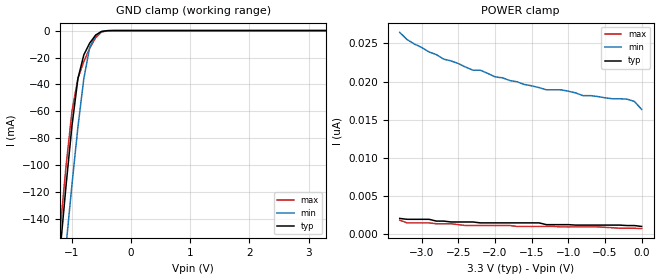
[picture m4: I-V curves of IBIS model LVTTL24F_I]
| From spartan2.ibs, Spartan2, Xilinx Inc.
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|   Model LVTTL24F_I
[Model]   LVTTL24F_I
Model_type   Input
Polarity   Non-Inverting
Vinl =   0.800V
Vinh =   2.000V
C_comp   6.5000pF   5.0000pF   8.0000pF
[Temperature Range]   27.0000   100.0000   0.000
[Voltage Range]   3.3000V   3.0000V   3.6000V
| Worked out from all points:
|   GND clamp passes 1 mA (typ) near -0.51 V on its own axis
[GND_clamp]
| voltage   I(typ)   I(min)   I(max)
-3.3V     -1.286A    -1.273A    -1.29A
-1.3V     -213.2mA   -255.1mA   -198mA
-1.2V     -163mA     -206.8mA   -147.7mA
-1.1V     -114.8mA   -159.6mA   -100.3mA
-1V       -70.57mA   -114.1mA   -59.86mA
-900mV    -35.79mA   -71.75mA   -35.46mA
-800mV    -18.04mA   -35.69mA   -22.98mA
-700mV    -9.256mA   -12.38mA   -13.06mA
-600mV    -3.388mA   -3.468mA   -5.299mA
-500mV    -637.4uA   -792.4uA   -1.07mA
-300mV    -3.973uA   -15.32uA   -4.185uA
3.3V      1.048nA    17.64nA    698.5pA
[POWER_clamp]
| voltage   I(typ)   I(min)   I(max)
-3.3V     2.095nA    26.43nA    1.863nA
-3.2V     1.979nA    25.49nA    1.513nA
-2.9V     1.979nA    23.87nA    1.513nA
-2.3V     1.63nA     21.48nA    1.164nA
-2.2V     1.513nA    21.48nA    1.164nA
-2V       1.513nA    20.61nA    1.164nA
-1.3V     1.281nA    18.92nA    1.048nA
-1.1V     1.281nA    18.92nA    989.5pA
-800mV    1.222nA    18.16nA    989.5pA
-200mV    1.164nA    17.7nA     814.9pA
-100mV    1.164nA    17.4nA     814.9pA
0V        1.048nA    16.36nA    756.7pA
